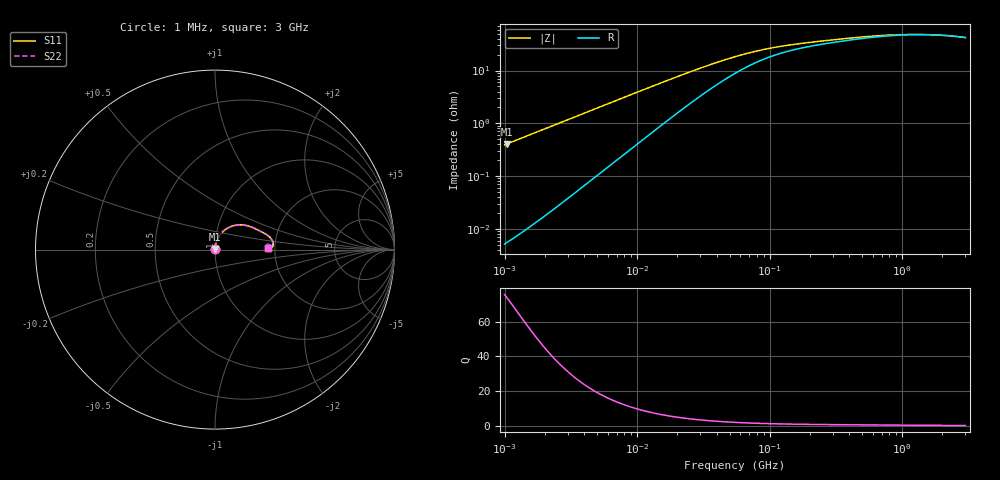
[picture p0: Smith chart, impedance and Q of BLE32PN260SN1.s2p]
! BLE32PN260SN1
# Hz S RI R 50
!Freq.(Hz) S11(Real) S11(Imag) S21(Real) S21(Imag) S12(Real) S12(Imag) S22(Real) S22(Imag)
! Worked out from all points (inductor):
!   401 points, 1 MHz to 3 GHz, reference 50 ohm
!   read as one part in series: L = 62.2 nH near 1.041 MHz
!   highest Q = 73.9 at 1.041 MHz (marker M1), where L = 62.2 nH
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1000000  6.7e-05 0.00391  0.9999 -0.00391  0.9999 -0.00391  6.7e-05 0.00391
1040844  7.16e-05 0.00407  0.9999 -0.00407  0.9999 -0.00407  7.16e-05 0.00407
3823119  0.000827 0.0149  0.9992 -0.0149  0.9992 -0.0149  0.000827 0.0149
7858845  0.00342 0.0303  0.9966 -0.0303  0.9966 -0.0303  0.00342 0.0303
1.461624e7  0.0114 0.0547  0.9886 -0.0547  0.9886 -0.0547  0.0114 0.0547
2.181181e7  0.0241 0.0775  0.9759 -0.0775  0.9759 -0.0775  0.0241 0.0775
3.065274e7  0.0435 0.1001  0.9565 -0.1001  0.9565 -0.1001  0.0435 0.1001
4.138676e7  0.0694 0.1192  0.9306 -0.1192  0.9306 -0.1192  0.0694 0.1192
5.477226e7  0.1007 0.1324  0.8993 -0.1324  0.8993 -0.1324  0.1007 0.1324
6.301011e7  0.1182 0.1362  0.8818 -0.1362  0.8818 -0.1362  0.1182 0.1362
7.248696e7  0.136 0.1379  0.864 -0.1379  0.864 -0.1379  0.136 0.1379
8.338914e7  0.1536 0.1375  0.8464 -0.1375  0.8464 -0.1375  0.1536 0.1375
9.787053e7  0.1728 0.1347  0.8272 -0.1347  0.8272 -0.1347  0.1728 0.1347
1.375402e8  0.2081 0.1238  0.7919 -0.1238  0.7919 -0.1238  0.2081 0.1238
2.094008e8  0.2419 0.108  0.7581 -0.108  0.7581 -0.108  0.2419 0.108
4.570858e8  0.2922 0.08  0.7078 -0.08  0.7078 -0.08  0.2922 0.08
6.049187e8  0.3068 0.0676  0.6932 -0.0676  0.6932 -0.0676  0.3068 0.0676
8.005644e8  0.3175 0.0538  0.6825 -0.0538  0.6825 -0.0538  0.3175 0.0538
1.147801e9  0.3245 0.0361  0.6755 -0.0361  0.6755 -0.0361  0.3245 0.0361
1.645649e9  0.3231 0.0208  0.6769 -0.0208  0.6769 -0.0208  0.3231 0.0208
2.221924e9  0.3144 0.0116  0.6856 -0.0116  0.6856 -0.0116  0.3144 0.0116
3e9  0.2969 0.00927  0.7031 -0.00927  0.7031 -0.00927  0.2969 0.00927
